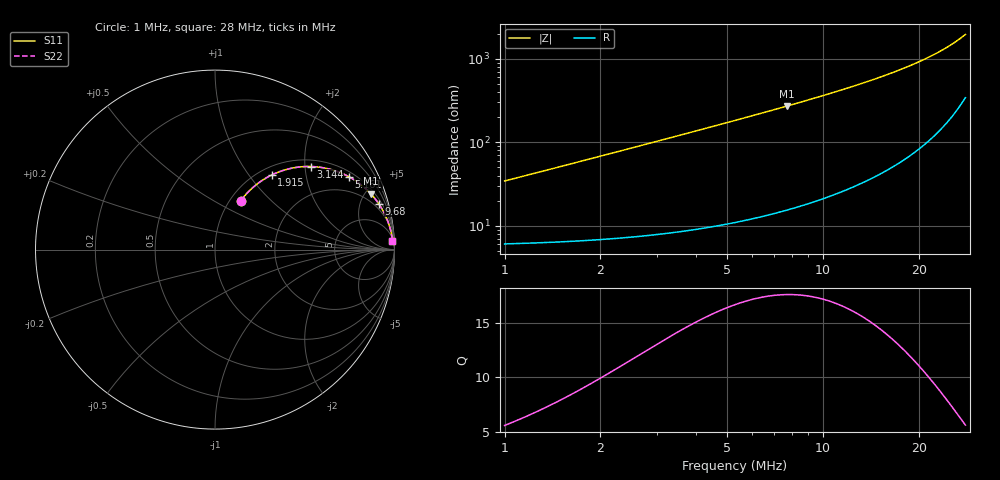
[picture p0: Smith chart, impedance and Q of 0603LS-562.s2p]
# MHz S MA R 50
!Freq  MagS11  AngS11  MagS21  AngS21  MagS12  AngS12  MagS22  AngS22
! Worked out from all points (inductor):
!   801 points, 1 MHz to 28 MHz, reference 50 ohm
!   read as one part in series: L = 5.39 uH near 1.017 MHz
!   highest Q = 17.6 at 7.698 MHz (marker M1), where L = 5.6 uH
!   S11 on the Smith chart (normalised r, x): 1 MHz: 1.12, +0.68; 1.915 MHz: 1.14, +1.30; 3.144 MHz: 1.16, +2.14; 5.161 MHz: 1.21, +3.56; 9.68 MHz: 1.40, +6.98; 28 MHz: 8, +39
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1  0.3092 62.1  0.8981 -17.7  0.8981 -17.7  0.3092 62.1
1.211188  0.3646 60.3  0.8783 -21.1  0.8783 -21.1  0.3646 60.3
1.418899  0.4157 58.1  0.8567 -24.3  0.8567 -24.3  0.4157 58.1
1.655323  0.4694 55.6  0.8304 -27.8  0.8304 -27.8  0.4694 55.6
1.915119  0.5228 52.7  0.8001 -31.3  0.8001 -31.3  0.5228 52.7
2.188175  0.573 49.8  0.7676 -34.8  0.7676 -34.8  0.573 49.8
2.479423  0.6201 46.9  0.733 -38.2  0.733 -38.2  0.6201 46.9
3.143841  0.7062 41.0  0.6574 -44.8  0.6574 -44.8  0.7062 41.0
3.622136  0.7533 37.3  0.6076 -48.7  0.6076 -48.7  0.7533 37.3
4.104244  0.7912 34.1  0.562 -52.1  0.562 -52.1  0.7912 34.1
4.611941  0.8231 31.2  0.5189 -55.2  0.5189 -55.2  0.8231 31.2
5.160899  0.8504 28.5  0.4774 -58.1  0.4774 -58.1  0.8504 28.5
5.516562  0.865 26.9  0.4532 -59.7  0.4532 -59.7  0.865 26.9
6.51668  0.8966 23.2  0.3945 -63.5  0.3945 -63.5  0.8966 23.2
7.698113  0.9216 19.8  0.3394 -66.9  0.3394 -66.9  0.9216 19.8
9.680023  0.9471 15.7  0.2708 -71.0  0.2708 -71.0  0.9471 15.7
10.00802  0.9501 15.1  0.2616 -71.5  0.2616 -71.5  0.9501 15.1
12.12159  0.9643 12.2  0.212 -74.3  0.212 -74.3  0.9643 12.2
14.55973  0.9741 9.8  0.1698 -76.4  0.1698 -76.4  0.9741 9.8
19.00754  0.9834 6.6  0.1162 -78.5  0.1162 -78.5  0.9834 6.6
23.50619  0.9878 4.5  0.07876 -78.9  0.07876 -78.9  0.9878 4.5
28  0.9899 2.9  0.05051 -77.1  0.05051 -77.1  0.9899 2.9
